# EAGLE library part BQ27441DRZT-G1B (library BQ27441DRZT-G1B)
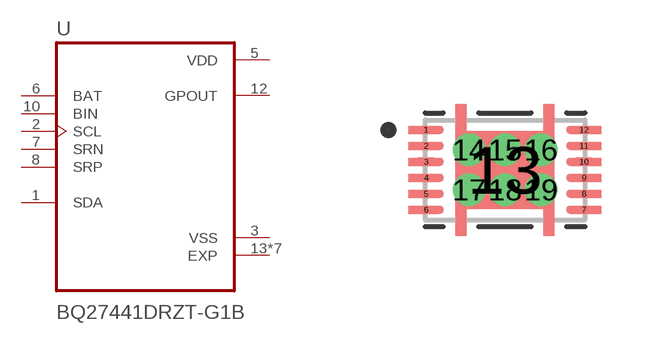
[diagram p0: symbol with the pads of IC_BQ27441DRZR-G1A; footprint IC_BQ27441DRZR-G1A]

Designator prefix U

## BQ27441DRZT-G1B  [IC_BQ27441DRZR-G1A]
1  SDA
2  SCL  in
3  VSS  pwr
5  VDD  pwr
6  BAT  in
7  SRN  in
8  SRP  in
10  BIN  in
12  GPOUT  out
13  EXP  pwr
14  EXP  pwr
15  EXP  pwr
16  EXP  pwr
17  EXP  pwr
18  EXP  pwr
19  EXP  pwr

## Footprint IC_BQ27441DRZR-G1A (pad centres in mm)
smd 0.4 x 0.2: 1 -1.975,1; 2 -1.975,0.6; 3 -1.975,0.2; 4 -1.975,-0.2; 5 -1.975,-0.6; 6 -1.975,-1; 7 1.975,-1; 8 1.975,-0.6; 9 1.975,-0.2; 10 1.975,0.2; 11 1.975,0.6; 12 1.975,1
smd 2.45 x 1.95: 13 0,0
drill 0.3 pad 0.5: 14 -0.9,0.5; 15 0,0.5; 16 0.9,0.5; 17 -0.9,-0.5; 18 0,-0.5; 19 0.9,-0.5

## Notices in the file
This work is licensed under a Creative Commons Attribution-ShareAlike 4.0 International License (CC BY-SA) with Design Exception 1.0
